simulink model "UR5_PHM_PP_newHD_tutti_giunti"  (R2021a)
settings: Solver=ode14x  StartTime=0.0  StopTime=Sim.time  FixedStep=Sim.dt  MaxStep=Sim.dt  RelTol=1e-3  EnableMultiTasking=on
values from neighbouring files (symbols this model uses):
  alpha_n = 0.98*pi/180    (= 0.0171042266695)    [parameters.m]
  alpha_t = 30*pi/180    (= 0.523598775598)    [parameters.m]
  alpha_TTS = 0    [parameters.m]
  alpha_Tw_L = -6.9e-4    (= -0.00069)    [parameters.m]
  alpha_Tw_R = 3.9e-3    (= 0.0039)    [parameters.m]
  Beta_TTS = 0    [parameters.m]
  c1 = 1e-2    (= 0.01)    [parameters.m]
  c2 = 1e-2    (= 0.01)    [parameters.m]
  c3 = 1e-2    (= 0.01)    [parameters.m]
  c4 = 1e-2    (= 0.01)    [parameters.m]
  c5 = 1e-2    (= 0.01)    [parameters.m]
  c6 = 1e-2    (= 0.01)    [parameters.m]
  Cb1 = 1.8e3    (= 1800)    [parameters.m]
  Cb2 = 1.8e3    (= 1800)    [parameters.m]
  Cb3 = 1.8e3    (= 1800)    [parameters.m]
  Cb4 = 1.8e3    (= 1800)    [parameters.m]
  Cb5 = 1.8e3    (= 1800)    [parameters.m]
  Cb6 = 1.8e3    (= 1800)    [parameters.m]
  Cth_housing = 153.90    (= 153.9)    [parameters.m]
  Cth_w = 74.20    (= 74.2)    [parameters.m]
  dt_PP = 0.05    [parameters.m]
  Fric1 = [fc_1/2 1e1 fc_1 fv_1]    [parameters.m]
  Fric2 = [fc_2/2 1e1 fc_2 fv_2]    [parameters.m]
  Fric3 = [fc_3/2 1e1 fc_3 fv_3]    [parameters.m]
  Fric4 = [fc_4/2 1e1 fc_4 fv_4]    [parameters.m]
  Fric5 = [fc_5/2 1e1 fc_5 fv_5]    [parameters.m]
  Fric6 = [fc_6/2 1e1 fc_6 fv_6]    [parameters.m]
  Hth_housing = 0.30    (= 0.3)    [parameters.m]
  Hth_w = 1.14    [parameters.m]
  I_actual = I_actual(1:10,:)    [trajcutting.m]
  J_CS1 = 7.12e-5    (= 7.12e-05)    [parameters.m]
  J_CS2 = 7.12e-5    (= 7.12e-05)    [parameters.m]
  J_CS3 = 7.12e-5    (= 7.12e-05)    [parameters.m]
  J_CS4 = 6e-6    (= 6e-06)    [parameters.m]
  J_CS5 = 6e-6    (= 6e-06)    [parameters.m]
  J_CS6 = 6e-6    (= 6e-06)    [parameters.m]
  J_FS1 = 1.62e-7    (= 1.62e-07)    [parameters.m]
  J_FS2 = 1.62e-7    (= 1.62e-07)    [parameters.m]
  J_FS3 = 1.62e-7    (= 1.62e-07)    [parameters.m]
  J_FS4 = 4.97e-8    (= 4.97e-08)    [parameters.m]
  J_FS5 = 4.97e-8    (= 4.97e-08)    [parameters.m]
  J_FS6 = 4.97e-8    (= 4.97e-08)    [parameters.m]
  J_WG1 = 3.56e-5    (= 3.56e-05)    [parameters.m]
  J_WG2 = 3.56e-5    (= 3.56e-05)    [parameters.m]
  J_WG3 = 3.56e-5    (= 3.56e-05)    [parameters.m]
  J_WG4 = 3e-6    (= 3e-06)    [parameters.m]
  J_WG5 = 3e-6    (= 3e-06)    [parameters.m]
  J_WG6 = 3e-6    (= 3e-06)    [parameters.m]
  K_i = 1    [parameters.m]
  K_p = 1    [parameters.m]
  K_torsCS1 = 4.78e6    (= 4780000)    [parameters.m]
  K_torsCS2 = 4.78e6    (= 4780000)    [parameters.m]
  K_torsCS3 = 4.78e6    (= 4780000)    [parameters.m]
  K_torsCS4 = 1.06e6    (= 1060000)    [parameters.m]
  K_torsCS5 = 1.06e6    (= 1060000)    [parameters.m]
  K_torsCS6 = 1.06e6    (= 1060000)    [parameters.m]
  K_torsWG1 = 9.56e5    (= 956000)    [parameters.m]
  K_torsWG2 = 9.56e5    (= 956000)    [parameters.m]
  K_torsWG3 = 9.56e5    (= 956000)    [parameters.m]
  K_torsWG4 = 1.84e5    (= 184000)    [parameters.m]
  K_torsWG5 = 1.84e5    (= 184000)    [parameters.m]
  K_torsWG6 = 1.84e5    (= 184000)    [parameters.m]
  K_v = 1    [parameters.m]
  Kb1 = 0.51e8    (= 51000000)    [parameters.m]
  Kb2 = 0.51e8    (= 51000000)    [parameters.m]
  Kb3 = 0.51e8    (= 51000000)    [parameters.m]
  Kb4 = 1.98e7    (= 19800000)    [parameters.m]
  Kb5 = 1.98e7    (= 19800000)    [parameters.m]
  Kb6 = 1.98e7    (= 19800000)    [parameters.m]
  Km1 = 1.2e9    (= 1200000000)    [parameters.m]
  Km2 = 1.2e9    (= 1200000000)    [parameters.m]
  Km3 = 1.2e9    (= 1200000000)    [parameters.m]
  Km4 = 5.55e8    (= 555000000)    [parameters.m]
  Km5 = 5.55e8    (= 555000000)    [parameters.m]
  Km6 = 5.55e8    (= 555000000)    [parameters.m]
  Kt1 = 0.96e5    (= 96000)    [parameters.m]
  Kt2 = 0.96e5    (= 96000)    [parameters.m]
  Kt3 = 0.96e5    (= 96000)    [parameters.m]
  Kt4 = 1.15e4    (= 11500)    [parameters.m]
  Kt5 = 1.15e4    (= 11500)    [parameters.m]
  Kt6 = 1.15e4    (= 11500)    [parameters.m]
  L = Motor.L_2/2    [parameters.m]
  m2 = polyfit(Temp(:,2),pBn_UR5_f_Temp(:,2),1)    [parameters.m]
  mb2 = polyfit(Temp(:,8),pBn_UR5_f_Temp(:,8),1)    [parameters.m]
  pickTime = t_pick(traj)    [parameters.m]
  placeTime = t_place(traj)    [parameters.m]
  q0 = q_target(1,:)    [testlaw_PP.m]
  q_CS01 = x(6)    [parameters.m]
  q_CS02 = x(6)    [parameters.m]
  q_CS03 = x(6)    [parameters.m]
  q_CS04 = x(6)    [parameters.m]
  q_CS05 = x(6)    [parameters.m]
  q_CS06 = x(6)    [parameters.m]
  q_WG01 = x(1)    [parameters.m]
  q_WG02 = x(1)    [parameters.m]
  q_WG03 = x(1)    [parameters.m]
  q_WG04 = x(1)    [parameters.m]
  q_WG05 = x(1)    [parameters.m]
  q_WG06 = x(1)    [parameters.m]
  quant_i = [Motor.imax1 Motor.imax2      Motor.imax3 Motor.imax4 Motor.imax5 Motor.imax6]/2^16    [parameters.m]
  R = Motor.R_2/2    [parameters.m]
  rg1 = 0.028    [parameters.m]
  rg2 = 0.028    [parameters.m]
  rg3 = 0.028    [parameters.m]
  rg4 = 0.0155    [parameters.m]
  rg5 = 0.0155    [parameters.m]
  rg6 = 0.0155    [parameters.m]
  sigma_p = 444.29    [parameters.m]
  sigma_v = 2*pi*1000    (= 6283.18530718)    [parameters.m]
  stiff_red = 1    [parameters.m]
  T_0 = Sim.temp    [parameters.m]
  T_switch = 1e-4    (= 0.0001)    [parameters.m]
  tau_i = 1/(fc_i*2*pi)    (= 7.95774715459e-05)    [parameters.m]
  U_s = 48    [parameters.m]
  var_i = 1e-1*[.0167 .0184 .0144 .0016      .0011 .0007]    [parameters.m]
  var_p = 1e-6*[.0943 .3877      .3478 .5436 .3400 .2081]    [parameters.m]
  var_v = 1e-4*[.0738 .1452      .1564 .4623 .1824 .0917]    [parameters.m]
  Wf_TTS_0 = 0    [parameters.m]
  Wf_TTS_ONOFF = 0    [parameters.m]
  x2_01 = x(3)    [parameters.m]
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undefined symbols (not defined in the file or in its folder): deg, Driver1, Driver2, Driver3, Driver4, Driver5, Driver6, elseif, geom, Ground, J1, J2, J3, J4, J5, J6, kg, L1, L2, L3, L4, L5, L6, LINK0, LINK1, LINK2, LINK3, LINK4, LINK5, LINK6, m, Motor, N, payload, ROBOTIQ_FT, s, Sim, Tool, X, Y, Z
libraries: sm_lib x35, nesl_utility x30, simulink x23, simulink_extras x11, spsTriangleGeneratorLib x6
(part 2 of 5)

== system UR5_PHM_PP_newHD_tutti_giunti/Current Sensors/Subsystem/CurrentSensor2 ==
  qm2 : Inport
  i2 [a,b,c] : Inport  Port=2
  Demux1 : Demux  Outputs=3
  Mux1 : Mux  Inputs=3
  Noise : UniformRandomNumber  Minimum=-var_i(2)  Maximum=var_i(2)  SampleTime=1/50
  Park Trnasform : Subsystem
  "Quantizer " : Quantizer  QuantizationInterval=quant_i(2)
  Sum : Sum  Inputs=|++
  Transfer Fcn : TransferFcn  Numerator=[K_i]  Denominator=[tau_i 1]
  Transfer Fcn1 : TransferFcn  Numerator=[K_i]  Denominator=[tau_i 1]
  Transfer Fcn2 : TransferFcn  Numerator=[K_i]  Denominator=[tau_i 1]
  "Zero-Order Hold " : ZeroOrderHold  SampleTime=1e-6
  i2 [dq0] : Outport
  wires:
  i2 [a,b,c]/1 -> Demux1/1
  Park Trnasform/1(i[d,q,0]) -> i2 [dq0]/1
  qm2/1 -> Park Trnasform/2(qm2)
  Noise/1 -> Sum/2
  "Quantizer "/1 -> Park Trnasform/1(i[a,b,c])
  "Zero-Order Hold "/1 -> "Quantizer "/1
  Sum/1 -> "Zero-Order Hold "/1
  Mux1/1 -> Sum/1
  Demux1/1 -> Transfer Fcn/1
  Demux1/2 -> Transfer Fcn1/1
  Demux1/3 -> Transfer Fcn2/1
  Transfer Fcn/1 -> Mux1/1
  Transfer Fcn1/1 -> Mux1/2
  Transfer Fcn2/1 -> Mux1/3

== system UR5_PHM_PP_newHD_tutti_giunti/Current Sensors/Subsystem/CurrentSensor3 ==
  i3 : Inport
  Noise : UniformRandomNumber  Minimum=-var_i(3)  Maximum=var_i(3)  SampleTime=1/50
  "Quantizer " : Quantizer  QuantizationInterval=quant_i(3)
  Sum : Sum  Inputs=|++
  Transfer Fcn (with initial outputs) : simulink_extras/Additional Linear/Transfer Fcn (with initial outputs)  N=[K_i]  D=[tau_i 1]  Y0=I_actual(1,3)  U0=I_actual(1,3)
  "Zero-Order Hold " : ZeroOrderHold  SampleTime=1e-6
  i3FB : Outport
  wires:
  Noise/1 -> Sum/2
  "Quantizer "/1 -> i3FB/1
  "Zero-Order Hold "/1 -> "Quantizer "/1
  Sum/1 -> "Zero-Order Hold "/1
  Transfer Fcn (with initial outputs)/1 -> Sum/1
  i3/1 -> Transfer Fcn (with initial outputs)/1

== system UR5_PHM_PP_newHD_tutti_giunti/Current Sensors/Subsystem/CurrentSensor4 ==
  i4 : Inport
  Noise : UniformRandomNumber  Minimum=-var_i(4)  Maximum=var_i(4)  SampleTime=1/50
  "Quantizer " : Quantizer  QuantizationInterval=quant_i(4)
  Sum : Sum  Inputs=|++
  Transfer Fcn (with initial outputs) : simulink_extras/Additional Linear/Transfer Fcn (with initial outputs)  N=[K_i]  D=[tau_i 1]  Y0=I_actual(1,4)  U0=I_actual(1,4)
  "Zero-Order Hold " : ZeroOrderHold  SampleTime=1e-6
  i4FB : Outport
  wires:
  Noise/1 -> Sum/2
  "Quantizer "/1 -> i4FB/1
  "Zero-Order Hold "/1 -> "Quantizer "/1
  Sum/1 -> "Zero-Order Hold "/1
  Transfer Fcn (with initial outputs)/1 -> Sum/1
  i4/1 -> Transfer Fcn (with initial outputs)/1

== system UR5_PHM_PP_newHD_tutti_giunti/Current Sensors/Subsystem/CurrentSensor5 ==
  i5 : Inport
  Noise : UniformRandomNumber  Minimum=-var_i(5)  Maximum=var_i(5)  SampleTime=1/50
  "Quantizer " : Quantizer  QuantizationInterval=quant_i(5)
  Sum : Sum  Inputs=|++
  Transfer Fcn (with initial outputs) : simulink_extras/Additional Linear/Transfer Fcn (with initial outputs)  N=[K_i]  D=[tau_i 1]  Y0=I_actual(1,5)  U0=I_actual(1,5)
  "Zero-Order Hold " : ZeroOrderHold  SampleTime=1e-6
  i5FB : Outport
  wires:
  Noise/1 -> Sum/2
  "Quantizer "/1 -> i5FB/1
  "Zero-Order Hold "/1 -> "Quantizer "/1
  Sum/1 -> "Zero-Order Hold "/1
  Transfer Fcn (with initial outputs)/1 -> Sum/1
  i5/1 -> Transfer Fcn (with initial outputs)/1

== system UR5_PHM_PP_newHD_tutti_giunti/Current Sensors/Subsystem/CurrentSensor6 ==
  i6 : Inport
  Noise : UniformRandomNumber  Minimum=-var_i(6)  Maximum=var_i(6)  SampleTime=1/50
  "Quantizer " : Quantizer  QuantizationInterval=quant_i(6)
  Sum : Sum  Inputs=|++
  Transfer Fcn (with initial outputs) : simulink_extras/Additional Linear/Transfer Fcn (with initial outputs)  N=[K_i]  D=[tau_i 1]  Y0=I_actual(1,6)  U0=I_actual(1,6)
  "Zero-Order Hold " : ZeroOrderHold  SampleTime=1e-6
  i6FB : Outport
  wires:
  "Quantizer "/1 -> i6FB/1
  Noise/1 -> Sum/2
  "Zero-Order Hold "/1 -> "Quantizer "/1
  Sum/1 -> "Zero-Order Hold "/1
  Transfer Fcn (with initial outputs)/1 -> Sum/1
  i6/1 -> Transfer Fcn (with initial outputs)/1

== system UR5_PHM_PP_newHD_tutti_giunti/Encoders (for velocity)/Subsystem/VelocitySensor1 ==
  qdm1 : Inport
  Noise : UniformRandomNumber  Minimum=-var_v(1)  Maximum=var_v(1)  SampleTime=1/5
  "Quantizer " : Quantizer  QuantizationInterval=quant_v
  Sum : Sum  Inputs=|++
  Transfer Fcn2 : TransferFcn  Numerator=[K_v]  Denominator=[1/sigma_v^2 2*zeta_v/sigma_v 1]
  "Zero-Order Hold " : ZeroOrderHold  SampleTime=1e-6
  qdmFB : Outport
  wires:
  qdm1/1 -> Transfer Fcn2/1
  Noise/1 -> Sum/2
  "Quantizer "/1 -> qdmFB/1
  "Zero-Order Hold "/1 -> "Quantizer "/1
  Sum/1 -> "Zero-Order Hold "/1
  Transfer Fcn2/1 -> Sum/1

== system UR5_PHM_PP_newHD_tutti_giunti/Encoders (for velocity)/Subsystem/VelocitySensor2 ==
  qdm2 : Inport
  Noise : UniformRandomNumber  Minimum=-var_v(2)  Maximum=var_v(2)  SampleTime=1/5
  "Quantizer " : Quantizer  QuantizationInterval=quant_v
  Sum : Sum  Inputs=|++
  Transfer Fcn2 : TransferFcn  Numerator=[K_v]  Denominator=[1/sigma_v^2 2*zeta_v/sigma_v 1]
  "Zero-Order Hold " : ZeroOrderHold  SampleTime=1e-6
  qdmFB2 : Outport
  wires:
  Noise/1 -> Sum/2
  "Quantizer "/1 -> qdmFB2/1
  "Zero-Order Hold "/1 -> "Quantizer "/1
  Sum/1 -> "Zero-Order Hold "/1
  qdm2/1 -> Transfer Fcn2/1
  Transfer Fcn2/1 -> Sum/1

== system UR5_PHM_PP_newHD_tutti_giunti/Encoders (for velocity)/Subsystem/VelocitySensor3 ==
  qdm3 : Inport
  Noise : UniformRandomNumber  Minimum=-var_v(3)  Maximum=var_v(3)  SampleTime=1/5
  "Quantizer " : Quantizer  QuantizationInterval=quant_v
  Sum : Sum  Inputs=|++
  Transfer Fcn2 : TransferFcn  Numerator=[K_v]  Denominator=[1/sigma_v^2 2*zeta_v/sigma_v 1]
  "Zero-Order Hold " : ZeroOrderHold  SampleTime=1e-6
  qdm3FB : Outport
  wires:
  Noise/1 -> Sum/2
  "Quantizer "/1 -> qdm3FB/1
  "Zero-Order Hold "/1 -> "Quantizer "/1
  Sum/1 -> "Zero-Order Hold "/1
  Transfer Fcn2/1 -> Sum/1
  qdm3/1 -> Transfer Fcn2/1

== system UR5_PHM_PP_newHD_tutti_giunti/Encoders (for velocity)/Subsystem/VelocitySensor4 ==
  qdm4 : Inport
  Noise : UniformRandomNumber  Minimum=-var_v(4)  Maximum=var_v(4)  SampleTime=1/5
  "Quantizer " : Quantizer  QuantizationInterval=quant_v
  Sum : Sum  Inputs=|++
  Transfer Fcn2 : TransferFcn  Numerator=[K_v]  Denominator=[1/sigma_v^2 2*zeta_v/sigma_v 1]
  "Zero-Order Hold " : ZeroOrderHold  SampleTime=1e-6
  qdm4FB : Outport
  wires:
  Noise/1 -> Sum/2
  "Quantizer "/1 -> qdm4FB/1
  "Zero-Order Hold "/1 -> "Quantizer "/1
  Sum/1 -> "Zero-Order Hold "/1
  Transfer Fcn2/1 -> Sum/1
  qdm4/1 -> Transfer Fcn2/1

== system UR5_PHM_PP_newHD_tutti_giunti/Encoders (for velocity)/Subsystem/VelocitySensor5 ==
  qdm5 : Inport
  Noise : UniformRandomNumber  Minimum=-var_v(5)  Maximum=var_v(5)  SampleTime=1/5
  "Quantizer " : Quantizer  QuantizationInterval=quant_v
  Sum : Sum  Inputs=|++
  Transfer Fcn2 : TransferFcn  Numerator=[K_v]  Denominator=[1/sigma_v^2 2*zeta_v/sigma_v 1]
  "Zero-Order Hold " : ZeroOrderHold  SampleTime=1e-6
  qdm5FB : Outport
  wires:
  Noise/1 -> Sum/2
  "Quantizer "/1 -> qdm5FB/1
  "Zero-Order Hold "/1 -> "Quantizer "/1
  Sum/1 -> "Zero-Order Hold "/1
  Transfer Fcn2/1 -> Sum/1
  qdm5/1 -> Transfer Fcn2/1

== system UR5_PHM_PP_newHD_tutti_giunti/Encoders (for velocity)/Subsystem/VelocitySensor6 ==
  qdm6 : Inport
  Noise : UniformRandomNumber  Minimum=-var_v(6)  Maximum=var_v(6)  SampleTime=1/5
  "Quantizer " : Quantizer  QuantizationInterval=quant_v
  Sum : Sum  Inputs=|++
  Transfer Fcn2 : TransferFcn  Numerator=[K_v]  Denominator=[1/sigma_v^2 2*zeta_v/sigma_v 1]
  "Zero-Order Hold " : ZeroOrderHold  SampleTime=1e-6
  qdm6FB : Outport
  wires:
  Noise/1 -> Sum/2
  "Quantizer "/1 -> qdm6FB/1
  "Zero-Order Hold "/1 -> "Quantizer "/1
  Sum/1 -> "Zero-Order Hold "/1
  Transfer Fcn2/1 -> Sum/1
  qdm6/1 -> Transfer Fcn2/1

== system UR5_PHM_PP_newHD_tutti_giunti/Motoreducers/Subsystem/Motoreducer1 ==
  q,qd,qdd : Inport
  Vset : Inport  Port=2
  DC Monophase Motor : Subsystem
  Demux : Demux  Outputs=3
  Demux1 : Demux  Outputs=3
  Gain : Gain  Gain=Motor.tau
  Gain1 : Gain  Gain=Motor.tau
  Gearbox : Subsystem
  New Gearbox's model : Subsystem
  Sum : Sum  Inputs=-+|
  Sum1 : Sum  Inputs=-+|
  Terminator : Terminator
  Terminator1 : Terminator
  Tu : Outport
  i : Outport  Port=2
  qm,qdm,qddm : Outport  Port=3
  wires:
  New Gearbox's model/2(C2) -> Gearbox/1(C)
  Sum1/1 -> New Gearbox's model/3(Delta_qd)
  Gain1/1 -> Sum1/1
  DC Monophase Motor/2(qm,qdm,qddm) -> qm,qdm,qddm/1, Demux/1
  Sum/1 -> New Gearbox's model/1(Delta_q)
  Demux/2 -> New Gearbox's model/4(qdm), Sum1/2
  Demux/3 -> Terminator1/1
  Demux1/1 -> [q], Gain/1
  Demux1/3 -> Terminator/1
  DC Monophase Motor/1(i) -> i/1
  Demux/1 -> Sum/2, New Gearbox's model/2(qm)
  Demux1/2 -> [qd], Gain1/1
  Vset/1 -> DC Monophase Motor/1(Vset)
  Gearbox/1(Tu) -> Tu/1  "Tu_j1"
  Gain/1 -> Sum/1
  q,qd,qdd/1 -> Demux1/1
  [qd] -> Gearbox/2(qd)
  [q] -> New Gearbox's model/5(q)
  [qd] -> New Gearbox's model/6(qd)
  New Gearbox's model/1(C1) -> DC Monophase Motor/2(C)

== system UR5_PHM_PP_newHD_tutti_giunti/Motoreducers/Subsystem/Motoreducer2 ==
  q,qd,qdd : Inport
  Vset : Inport  Port=2
  BLAC : Subsystem
  Constant : Constant  Value=Sim.temp
  Demux : Demux  Outputs=3
  Demux1 : Demux  Outputs=3
  Gain : Gain  Gain=Motor.tau
  Gain1 : Gain  Gain=Motor.tau
  Gearbox : Subsystem
  New Gearbox's Model : Subsystem
  Scope : Scope
  Scope1 : Scope
  Sum : Sum  Inputs=-+|
  Sum1 : Sum  Inputs=-+|
  Terminator : Terminator
  Terminator1 : Terminator
  Windings temperature : Subsystem
  Tu : Outport
  i[a.b.c] : Outport  Port=2
  qm,qdm,qddm : Outport  Port=3
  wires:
  Windings temperature/1(Tw [°C]) -> BLAC/2(T_w [°C])
  BLAC/3(W_joule[W]) -> Windings temperature/1(W_joule [W])
  Vset/1 -> BLAC/1(V[ao,bo,co])
  Constant/1 -> Windings temperature/2(T_ext [°C])
  BLAC/1(i[a,b,c]) -> i[a.b.c]/1
  q,qd,qdd/1 -> Demux1/1
  Demux1/2 -> [qd], Gain1/1
  Demux1/3 -> Terminator/1
  Gain1/1 -> Sum1/1
  BLAC/2(qm,qdm,qddm) -> Demux/1, qm,qdm,qddm/1
  Demux/1 -> New Gearbox's Model/2(qm), Sum/2
  Gain/1 -> Sum/1
  Sum/1 -> Scope/1, New Gearbox's Model/1(Delta_q)  "Delta_q_j2"
  Sum1/1 -> New Gearbox's Model/3(Delta_qd)
  Demux/3 -> Terminator1/1
  Demux/2 -> New Gearbox's Model/4(qdm), Sum1/2
  Demux1/1 -> [q], Gain/1
  [qd] -> Gearbox/2(qd)
  Gearbox/1(Tu) -> Tu/1  "Tu_j2"
  Windings temperature/2(Th [°C]) -> Gearbox/3(Th [°C])
  New Gearbox's Model/2(C2) -> Scope1/1, Gearbox/1(C)
  [q] -> New Gearbox's Model/5(q)
  New Gearbox's Model/1(C1) -> BLAC/3(C)
  [qd] -> New Gearbox's Model/6(qd)

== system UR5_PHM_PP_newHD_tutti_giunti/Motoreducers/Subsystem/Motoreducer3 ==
  q,qd,qdd : Inport
  Vset : Inport  Port=2
  DC Monophase Motor3 : Subsystem
  Demux4 : Demux  Outputs=3
  Demux5 : Demux  Outputs=3
  Gain4 : Gain  Gain=Motor.tau
  Gain5 : Gain  Gain=Motor.tau
  Gearbox3 : Subsystem
  New Gearbox's Model : Subsystem
  Sum4 : Sum  Inputs=-+|
  Sum5 : Sum  Inputs=-+|
  Terminator4 : Terminator
  Terminator5 : Terminator
  Tu : Outport
  i : Outport  Port=2
  qm,qdm,qddm : Outport  Port=3
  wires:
  Gain4/1 -> Sum4/1
  Sum5/1 -> New Gearbox's Model/4(Delta_qd)
  New Gearbox's Model/2(Tu) -> Gearbox3/1(C)
  DC Monophase Motor3/2(qm,qdm,qddm) -> qm,qdm,qddm/1, Demux4/1
  Demux5/3 -> Terminator4/1
  Demux5/2 -> [qd], Gain5/1
  Demux4/2 -> New Gearbox's Model/3(qdm), Sum5/2
  Demux4/3 -> Terminator5/1
  Sum4/1 -> New Gearbox's Model/1(Delta_q)
  [qd] -> Gearbox3/2(qd)
  DC Monophase Motor3/1(i) -> i/1
  Demux5/1 -> [q], Gain4/1
  Vset/1 -> DC Monophase Motor3/1(Vset)
  q,qd,qdd/1 -> Demux5/1
  Gain5/1 -> Sum5/1
  Gearbox3/1(Tu) -> Tu/1  "Tu_j3"
  Demux4/1 -> New Gearbox's Model/2(qm), Sum4/2
  [q] -> New Gearbox's Model/5(q)
  [qd] -> New Gearbox's Model/6(qd)
  New Gearbox's Model/1(C1) -> DC Monophase Motor3/2(C)

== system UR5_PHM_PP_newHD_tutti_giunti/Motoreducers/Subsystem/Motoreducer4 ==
  q,qd,qdd : Inport
  Vset : Inport  Port=2
  DC Monophase Motor4 : Subsystem
  Demux6 : Demux  Outputs=3
  Demux7 : Demux  Outputs=3
  Gain6 : Gain  Gain=Motor.tau
  Gain7 : Gain  Gain=Motor.tau
  Gearbox4 : Subsystem
  New Gearbox's Model : Subsystem
  Sum6 : Sum  Inputs=-+|
  Sum7 : Sum  Inputs=-+|
  Terminator6 : Terminator
  Terminator7 : Terminator
  Tu : Outport
  i : Outport  Port=2
  qm,qdm,qddm : Outport  Port=3
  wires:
  Demux7/2 -> [qd], Gain7/1
  DC Monophase Motor4/2(qm,qdm,qddm) -> qm,qdm,qddm/1, Demux6/1
  Gain7/1 -> Sum7/1
  Sum6/1 -> New Gearbox's Model/1(Delta_q)
  [qd] -> Gearbox4/2(qd)
  Demux6/2 -> New Gearbox's Model/3(qdm), Sum7/2
  New Gearbox's Model/2(C2) -> Gearbox4/1(C)
  Gain6/1 -> Sum6/1
  Demux7/3 -> Terminator6/1
  Demux6/1 -> New Gearbox's Model/2(qm), Sum6/2
  Demux7/1 -> Gain6/1, [q]
  DC Monophase Motor4/1(i) -> i/1
  Sum7/1 -> New Gearbox's Model/4(Delta_qd)
  q,qd,qdd/1 -> Demux7/1
  Vset/1 -> DC Monophase Motor4/1(Vset)
  Demux6/3 -> Terminator7/1
  Gearbox4/1(Tu) -> Tu/1  "Tu_j4"
  [q] -> New Gearbox's Model/5(q)
  [qd] -> New Gearbox's Model/6(qd)
  New Gearbox's Model/1(C1) -> DC Monophase Motor4/2(C)

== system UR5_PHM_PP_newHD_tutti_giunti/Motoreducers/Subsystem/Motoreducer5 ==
  q,qd,qdd : Inport
  Vset : Inport  Port=2
  DC Monophase Motor5 : Subsystem
  Demux8 : Demux  Outputs=3
  Demux9 : Demux  Outputs=3
  Gain8 : Gain  Gain=Motor.tau
  Gain9 : Gain  Gain=Motor.tau
  Gearbox5 : Subsystem
  New Gearbox's Model : Subsystem
  Sum8 : Sum  Inputs=-+|
  Sum9 : Sum  Inputs=-+|
  Terminator8 : Terminator
  Terminator9 : Terminator
  Tu : Outport
  i : Outport  Port=2
  qm,qdm,qddm : Outport  Port=3
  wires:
  Demux9/3 -> Terminator8/1
  Demux8/1 -> New Gearbox's Model/2(qm), Sum8/2
  Gain8/1 -> Sum8/1
  New Gearbox's Model/2(C2) -> Gearbox5/1(C)
  Demux8/3 -> Terminator9/1
  Demux8/2 -> New Gearbox's Model/3(qdm), Sum9/2
  Gain9/1 -> Sum9/1
  Sum9/1 -> New Gearbox's Model/4(Delta_qd)
  Sum8/1 -> New Gearbox's Model/1(Delta_q)
  Demux9/1 -> [q], Gain8/1
  Vset/1 -> DC Monophase Motor5/1(Vset)
  Demux9/2 -> [qd], Gain9/1
  DC Monophase Motor5/2(qm,qdm,qddm) -> qm,qdm,qddm/1, Demux8/1
  q,qd,qdd/1 -> Demux9/1
  [qd] -> Gearbox5/2(qd)
  DC Monophase Motor5/1(i) -> i/1
  Gearbox5/1(Tu) -> Tu/1  "Tu_j5"
  [q] -> New Gearbox's Model/5(q)
  [qd] -> New Gearbox's Model/6(qd)
  New Gearbox's Model/1(C1) -> DC Monophase Motor5/2(C)

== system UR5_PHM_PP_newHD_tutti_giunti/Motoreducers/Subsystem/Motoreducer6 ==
  q,qd,qdd : Inport
  Vset : Inport  Port=2
  DC Monophase Motor6 : Subsystem
  Demux10 : Demux  Outputs=3
  Demux11 : Demux  Outputs=3
  Gain10 : Gain  Gain=Motor.tau
  Gain11 : Gain  Gain=Motor.tau
  Gearbox6 : Subsystem
  New  Gearbox's Model : Subsystem
  Sum10 : Sum  Inputs=-+|
  Sum11 : Sum  Inputs=-+|
  Terminator10 : Terminator
  Terminator11 : Terminator
  Tu : Outport
  i : Outport  Port=2
  qm,qdm,qddm : Outport  Port=3
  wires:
  Vset/1 -> DC Monophase Motor6/1(Vset)
  q,qd,qdd/1 -> Demux11/1
  DC Monophase Motor6/1(i) -> i/1
  Demux11/1 -> Gain10/1, [q]
  Gain10/1 -> Sum10/1
  Demux10/1 -> New  Gearbox's Model/2(qm), Sum10/2
  Demux11/2 -> [qd], Gain11/1
  Sum11/1 -> New  Gearbox's Model/4(Delta_qd)
  [qd] -> Gearbox6/2(qd)
  Sum10/1 -> New  Gearbox's Model/1(Delta_q)
  Demux10/2 -> New  Gearbox's Model/3(qdm), Sum11/2
  Demux10/3 -> Terminator11/1
  New  Gearbox's Model/2(C2) -> Gearbox6/1(C)
  DC Monophase Motor6/2(qm,qdm,qddm) -> qm,qdm,qddm/1, Demux10/1
  Demux11/3 -> Terminator10/1
  Gain11/1 -> Sum11/1
  Gearbox6/1(Tu) -> Tu/1  "Tu_j6"
  [q] -> New  Gearbox's Model/5(q)
  [qd] -> New  Gearbox's Model/6(qd)
  New  Gearbox's Model/1(C1) -> DC Monophase Motor6/2(C)

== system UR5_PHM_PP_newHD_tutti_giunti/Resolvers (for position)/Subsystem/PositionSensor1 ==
  q1 : Inport
  Noise : UniformRandomNumber  Minimum=-var_p(1)  Maximum=var_p(1)  SampleTime=1/4
  "Quantizer " : Quantizer  QuantizationInterval=quant_p
  Sum : Sum  Inputs=|++
  Transfer Fcn (with initial outputs)2 : simulink_extras/Additional Linear/Transfer Fcn (with initial outputs)  N=[K_p]  D=[1/sigma_p^2 2*zeta_p/sigma_p 1]  Y0=q0(1)  U0=q0(1)
  "Zero-Order Hold " : ZeroOrderHold  SampleTime=1e-6
  q1FB : Outport
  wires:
  Noise/1 -> Sum/2
  "Quantizer "/1 -> q1FB/1
  "Zero-Order Hold "/1 -> "Quantizer "/1
  Sum/1 -> "Zero-Order Hold "/1
  Transfer Fcn (with initial outputs)2/1 -> Sum/1
  q1/1 -> Transfer Fcn (with initial outputs)2/1

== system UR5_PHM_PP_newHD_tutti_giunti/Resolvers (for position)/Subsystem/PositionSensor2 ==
  q2 : Inport
  Noise : UniformRandomNumber  Minimum=-var_p(2)  Maximum=var_p(2)  SampleTime=1/4
  "Quantizer " : Quantizer  QuantizationInterval=quant_p
  Sum : Sum  Inputs=|++
  Transfer Fcn (with initial outputs)2 : simulink_extras/Additional Linear/Transfer Fcn (with initial outputs)  N=[K_p]  D=[1/sigma_p^2 2*zeta_p/sigma_p 1]  Y0=q0(2)  U0=q0(2)
  "Zero-Order Hold " : ZeroOrderHold  SampleTime=1e-6
  q2FB : Outport
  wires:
  "Quantizer "/1 -> q2FB/1
  "Zero-Order Hold "/1 -> "Quantizer "/1
  Sum/1 -> "Zero-Order Hold "/1
  Transfer Fcn (with initial outputs)2/1 -> Sum/1
  q2/1 -> Transfer Fcn (with initial outputs)2/1
  Noise/1 -> Sum/2

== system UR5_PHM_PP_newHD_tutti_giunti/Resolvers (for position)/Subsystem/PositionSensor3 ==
  q3 : Inport
  Noise : UniformRandomNumber  Minimum=-var_p(3)  Maximum=var_p(3)  SampleTime=1/4
  "Quantizer " : Quantizer  QuantizationInterval=quant_p
  Sum : Sum  Inputs=|++
  Transfer Fcn (with initial outputs)2 : simulink_extras/Additional Linear/Transfer Fcn (with initial outputs)  N=[K_p]  D=[1/sigma_p^2 2*zeta_p/sigma_p 1]  Y0=q0(3)  U0=q0(3)
  "Zero-Order Hold " : ZeroOrderHold  SampleTime=1e-6
  q3FB : Outport
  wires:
  Sum/1 -> "Zero-Order Hold "/1
  "Zero-Order Hold "/1 -> "Quantizer "/1
  "Quantizer "/1 -> q3FB/1
  Noise/1 -> Sum/2
  q3/1 -> Transfer Fcn (with initial outputs)2/1
  Transfer Fcn (with initial outputs)2/1 -> Sum/1

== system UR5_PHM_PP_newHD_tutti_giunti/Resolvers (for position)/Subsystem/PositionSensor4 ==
  q4 : Inport
  Noise : UniformRandomNumber  Minimum=-var_p(4)  Maximum=var_p(4)  SampleTime=1/4
  "Quantizer " : Quantizer  QuantizationInterval=quant_p
  Sum : Sum  Inputs=|++
  Transfer Fcn (with initial outputs)2 : simulink_extras/Additional Linear/Transfer Fcn (with initial outputs)  N=[K_p]  D=[1/sigma_p^2 2*zeta_p/sigma_p 1]  Y0=q0(4)  U0=q0(4)
  "Zero-Order Hold " : ZeroOrderHold  SampleTime=1e-6
  q4FB : Outport
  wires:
  Noise/1 -> Sum/2
  "Quantizer "/1 -> q4FB/1
  "Zero-Order Hold "/1 -> "Quantizer "/1
  Sum/1 -> "Zero-Order Hold "/1
  q4/1 -> Transfer Fcn (with initial outputs)2/1
  Transfer Fcn (with initial outputs)2/1 -> Sum/1

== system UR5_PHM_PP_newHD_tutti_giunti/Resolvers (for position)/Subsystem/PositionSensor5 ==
  q5 : Inport
  Noise : UniformRandomNumber  Minimum=-var_p(5)  Maximum=var_p(5)  SampleTime=1/4
  "Quantizer " : Quantizer  QuantizationInterval=quant_p
  Sum : Sum  Inputs=|++
  Transfer Fcn (with initial outputs)2 : simulink_extras/Additional Linear/Transfer Fcn (with initial outputs)  N=[K_p]  D=[1/sigma_p^2 2*zeta_p/sigma_p 1]  Y0=q0(5)  U0=q0(5)
  "Zero-Order Hold " : ZeroOrderHold  SampleTime=1e-6
  q5FB : Outport
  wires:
  Sum/1 -> "Zero-Order Hold "/1
  "Zero-Order Hold "/1 -> "Quantizer "/1
  "Quantizer "/1 -> q5FB/1
  Noise/1 -> Sum/2
  q5/1 -> Transfer Fcn (with initial outputs)2/1
  Transfer Fcn (with initial outputs)2/1 -> Sum/1

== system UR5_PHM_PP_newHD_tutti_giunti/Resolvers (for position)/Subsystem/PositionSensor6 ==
  q6 : Inport
  Noise : UniformRandomNumber  Minimum=-var_p(6)  Maximum=var_p(6)  SampleTime=1/4
  "Quantizer " : Quantizer  QuantizationInterval=quant_p
  Sum : Sum  Inputs=|++
  Transfer Fcn (with initial outputs)2 : simulink_extras/Additional Linear/Transfer Fcn (with initial outputs)  N=[K_p]  D=[1/sigma_p^2 2*zeta_p/sigma_p 1]  Y0=q0(6)  U0=q0(6)
  "Zero-Order Hold " : ZeroOrderHold  SampleTime=1e-6
  q6FB : Outport
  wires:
  Noise/1 -> Sum/2
  "Quantizer "/1 -> q6FB/1
  "Zero-Order Hold "/1 -> "Quantizer "/1
  Sum/1 -> "Zero-Order Hold "/1
  Transfer Fcn (with initial outputs)2/1 -> Sum/1
  q6/1 -> Transfer Fcn (with initial outputs)2/1

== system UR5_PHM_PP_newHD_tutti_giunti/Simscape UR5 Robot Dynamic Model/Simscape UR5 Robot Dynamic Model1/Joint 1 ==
  T1 : Inport
  A_01*E_01 : sm_lib/Frames and Transforms/Rigid Transform  TranslationMethod=None  TranslationStandardOffset=0  TranslationLengthUnit=mm  TranslationStandardAxis=+Z  TranslationCartesianOffset=A01t  TranslationROffset=0  TranslationROffsetUnits=m  TranslationZOffset=0  TranslationZOffsetUnits=m  TranslationThetaOffset=0  TranslationThetaOffsetUnits=deg  RotationMethod=RotationMatrix  RotationAngleUnits=deg  RotationStandardAxis=+Z  RotationAngle=0.0  RotationArbitraryAxis=[0 0 1]  FollAlignAxisA=+X  BaseAlignAxisA=+Y  FollAlignAxisB=+Y  BaseAlignAxisB=+Z  RotationSequenceAxes=FollowerAxes  RotationSequence=XYX  RotationSequenceAngles=[0 0 0]  RotationSequenceAnglesUnits=deg  RotationMatrix=A01r
  A_01*E_1 : sm_lib/Frames and Transforms/Rigid Transform  TranslationMethod=Cartesian  TranslationStandardOffset=0  TranslationLengthUnit=mm  TranslationStandardAxis=+Z  TranslationCartesianOffset=A01t  TranslationROffset=0  TranslationROffsetUnits=m  TranslationZOffset=0  TranslationZOffsetUnits=m  TranslationThetaOffset=0  TranslationThetaOffsetUnits=deg  RotationMethod=None  RotationAngleUnits=deg  RotationStandardAxis=+Z  RotationAngle=0.0  RotationArbitraryAxis=[0 0 1]  FollAlignAxisA=+X  BaseAlignAxisA=+Y  FollAlignAxisB=+Y  BaseAlignAxisB=+Z  RotationSequenceAxes=FollowerAxes  RotationSequence=XYX  RotationSequenceAngles=[0 0 0]  RotationSequenceAnglesUnits=deg  RotationMatrix=A01r
  Mux : Mux  Inputs=3
  PS-Simulink Converter1 : nesl_utility/PS-Simulink Converter  PhysicalDomain=network_engine_domain  SubClassName=ps_output  LeftPortType=input  RightPortType=output  PseudoPeriodic=off  Frequencies=[]  Unit=1  AffineConversion=off
  PS-Simulink Converter2 : nesl_utility/PS-Simulink Converter  PhysicalDomain=network_engine_domain  SubClassName=ps_output  LeftPortType=input  RightPortType=output  PseudoPeriodic=off  Frequencies=[]  Unit=1  AffineConversion=off
  PS-Simulink Converter7 : nesl_utility/PS-Simulink Converter  PhysicalDomain=network_engine_domain  SubClassName=ps_output  LeftPortType=input  RightPortType=output  PseudoPeriodic=off  Frequencies=[]  Unit=1  AffineConversion=off
  Revolute Joint1 : sm_lib/Joints/Revolute Joint  JointMode=Normal  SenseConstraintForce=off  SenseConstraintForceX=off  SenseConstraintForceY=off  SenseConstraintForceZ=off  SenseConstraintTorque=off  SenseConstraintTorqueX=off  SenseConstraintTorqueY=off  SenseConstraintTorqueZ=off  SenseTotalForce=off  SenseTotalForceX=off  SenseTotalForceY=off  SenseTotalForceZ=off  SenseTotalTorque=off  SenseTotalTorqueX=off  SenseTotalTorqueY=off  SenseTotalTorqueZ=off  CompositeWrenchDir=FollowerOnBase  CompositeWrenchFrame=BaseFrame  EquilibriumPosition=0  EquilibriumPositionUnits=deg  SpringStiffness=0  SpringStiffnessUnits=N*m/deg  DampingCoefficient=0  DampingCoefficientUnits=N*m/(deg/s)  TorqueActuationMode=InputTorque  MotionActuationMode=ComputedMotion  SensePosition=on  SenseVelocity=on  SenseAcceleration=on  SenseTorqueForce=off  SenseLowerLimitTorqueForce=off  SenseUpperLimitTorqueForce=off  LowerLimitSpecify=on  LowerLimitBound=-J1.al  LowerLimitBoundUnits=deg  LowerLimitStiffness=1e4  LowerLimitStiffnessUnits=N*m/deg  LowerLimitDamping=10  LowerLimitDampingUnits=N*m/(deg/s)  LowerLimitTransitionRegionWidth=0.1  LowerLimitTransitionRegionWidthUnits=deg  UpperLimitSpecify=on  UpperLimitBound=J1.al  UpperLimitBoundUnits=deg  UpperLimitStiffness=1e4  UpperLimitStiffnessUnits=N*m/deg  UpperLimitDamping=10  UpperLimitDampingUnits=N*m/(deg/s)  UpperLimitTransitionRegionWidth=0.1  UpperLimitTransitionRegionWidthUnits=deg  PositionTargetSpecify=on  PositionTargetPriority=Low  PositionTargetValue=q0(1)  PositionTargetValueUnits=rad  VelocityTargetSpecify=off  VelocityTargetPriority=High  VelocityTargetValue=0  VelocityTargetValueUnits=deg/s
  Simulink-PS Converter : nesl_utility/Simulink-PS Converter  PhysicalDomain=network_engine_domain  SubClassName=ps_input  LeftPortType=input  RightPortType=output  PseudoPeriodic=off  Frequencies=[]  NoiseDistribution=none  NoiseParameters=[]  Unit=1  AffineConversion=off  FilteringAndDerivatives=provide  SimscapeFilterOrder=1  InputFilterTimeConstant=0.001  UdotUserProvided=0
  Link 0 : PMIOPort  Side=Left
  Link 1 : PMIOPort  Port=2  Side=Right
  q1,qd1,qdd1 : Outport
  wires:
  T1/1 -> Simulink-PS Converter/1
  PS-Simulink Converter7/1 -> Mux/2
  Mux/1 -> q1,qd1,qdd1/1
  PS-Simulink Converter1/1 -> Mux/1
  PS-Simulink Converter2/1 -> Mux/3
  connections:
  Revolute Joint1/LConn1 -- A_01*E_1/RConn1
  A_01*E_1/LConn1 -- A_01*E_01/RConn1
  Revolute Joint1/RConn1 -- Link 1/RConn1
  Link 0/RConn1 -- A_01*E_01/LConn1
  Simulink-PS Converter/RConn1 -- Revolute Joint1/LConn2
  Revolute Joint1/RConn2 -- PS-Simulink Converter1/LConn1
  Revolute Joint1/RConn3 -- PS-Simulink Converter7/LConn1
  Revolute Joint1/RConn4 -- PS-Simulink Converter2/LConn1

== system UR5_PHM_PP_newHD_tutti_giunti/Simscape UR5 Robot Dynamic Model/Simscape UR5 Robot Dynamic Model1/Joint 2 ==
  T2 : Inport
  A_12*E_1 : sm_lib/Frames and Transforms/Rigid Transform  TranslationMethod=Cartesian  TranslationStandardOffset=0  TranslationLengthUnit=mm  TranslationStandardAxis=+Z  TranslationCartesianOffset=A12t  TranslationROffset=0  TranslationROffsetUnits=m  TranslationZOffset=0  TranslationZOffsetUnits=m  TranslationThetaOffset=0  TranslationThetaOffsetUnits=deg  RotationMethod=None  RotationAngleUnits=deg  RotationStandardAxis=+Z  RotationAngle=0.0  RotationArbitraryAxis=[0 0 1]  FollAlignAxisA=+X  BaseAlignAxisA=+Y  FollAlignAxisB=+Y  BaseAlignAxisB=+Z  RotationSequenceAxes=FollowerAxes  RotationSequence=XYX  RotationSequenceAngles=[0 0 0]  RotationSequenceAnglesUnits=deg  RotationMatrix=A12r
  A_12*E_12 : sm_lib/Frames and Transforms/Rigid Transform  TranslationMethod=None  TranslationStandardOffset=0  TranslationLengthUnit=mm  TranslationStandardAxis=+Z  TranslationCartesianOffset=A12t  TranslationROffset=0  TranslationROffsetUnits=m  TranslationZOffset=0  TranslationZOffsetUnits=m  TranslationThetaOffset=0  TranslationThetaOffsetUnits=deg  RotationMethod=RotationMatrix  RotationAngleUnits=deg  RotationStandardAxis=+Z  RotationAngle=0.0  RotationArbitraryAxis=[0 0 1]  FollAlignAxisA=+X  BaseAlignAxisA=+Y  FollAlignAxisB=+Y  BaseAlignAxisB=+Z  RotationSequenceAxes=FollowerAxes  RotationSequence=XYX  RotationSequenceAngles=[0 0 0]  RotationSequenceAnglesUnits=deg  RotationMatrix=A12r
  Mux : Mux  Inputs=3
  PS-Simulink Converter1 : nesl_utility/PS-Simulink Converter  PhysicalDomain=network_engine_domain  SubClassName=ps_output  LeftPortType=input  RightPortType=output  PseudoPeriodic=off  Frequencies=[]  Unit=1  AffineConversion=off
  PS-Simulink Converter2 : nesl_utility/PS-Simulink Converter  PhysicalDomain=network_engine_domain  SubClassName=ps_output  LeftPortType=input  RightPortType=output  PseudoPeriodic=off  Frequencies=[]  Unit=1  AffineConversion=off
  PS-Simulink Converter7 : nesl_utility/PS-Simulink Converter  PhysicalDomain=network_engine_domain  SubClassName=ps_output  LeftPortType=input  RightPortType=output  PseudoPeriodic=off  Frequencies=[]  Unit=1  AffineConversion=off
  Revolute Joint2 : sm_lib/Joints/Revolute Joint  JointMode=Normal  SenseConstraintForce=off  SenseConstraintForceX=off  SenseConstraintForceY=off  SenseConstraintForceZ=off  SenseConstraintTorque=off  SenseConstraintTorqueX=off  SenseConstraintTorqueY=off  SenseConstraintTorqueZ=off  SenseTotalForce=off  SenseTotalForceX=off  SenseTotalForceY=off  SenseTotalForceZ=off  SenseTotalTorque=off  SenseTotalTorqueX=off  SenseTotalTorqueY=off  SenseTotalTorqueZ=off  CompositeWrenchDir=FollowerOnBase  CompositeWrenchFrame=BaseFrame  EquilibriumPosition=0  EquilibriumPositionUnits=deg  SpringStiffness=0  SpringStiffnessUnits=N*m/deg  DampingCoefficient=0  DampingCoefficientUnits=N*m/(deg/s)  TorqueActuationMode=InputTorque  MotionActuationMode=ComputedMotion  SensePosition=on  SenseVelocity=on  SenseAcceleration=on  SenseTorqueForce=off  SenseLowerLimitTorqueForce=off  SenseUpperLimitTorqueForce=off  LowerLimitSpecify=on  LowerLimitBound=-J2.al  LowerLimitBoundUnits=deg  LowerLimitStiffness=1e4  LowerLimitStiffnessUnits=N*m/deg  LowerLimitDamping=10  LowerLimitDampingUnits=N*m/(deg/s)  LowerLimitTransitionRegionWidth=0.1  LowerLimitTransitionRegionWidthUnits=deg  UpperLimitSpecify=on  UpperLimitBound=J2.al  UpperLimitBoundUnits=deg  UpperLimitStiffness=1e4  UpperLimitStiffnessUnits=N*m/deg  UpperLimitDamping=10  UpperLimitDampingUnits=N*m/(deg/s)  UpperLimitTransitionRegionWidth=0.1  UpperLimitTransitionRegionWidthUnits=deg  PositionTargetSpecify=on  PositionTargetPriority=High  PositionTargetValue=q0(2)  PositionTargetValueUnits=rad  VelocityTargetSpecify=off  VelocityTargetPriority=High  VelocityTargetValue=0  VelocityTargetValueUnits=deg/s
  Simulink-PS Converter : nesl_utility/Simulink-PS Converter  PhysicalDomain=network_engine_domain  SubClassName=ps_input  LeftPortType=input  RightPortType=output  PseudoPeriodic=off  Frequencies=[]  NoiseDistribution=none  NoiseParameters=[]  Unit=1  AffineConversion=off  FilteringAndDerivatives=provide  SimscapeFilterOrder=1  InputFilterTimeConstant=0.001  UdotUserProvided=0
  Link 1 : PMIOPort  Side=Left
  Link 2 : PMIOPort  Port=2  Side=Right
  q2,qd2,qdd2 : Outport
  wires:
  PS-Simulink Converter1/1 -> Mux/1
  T2/1 -> Simulink-PS Converter/1
  Mux/1 -> q2,qd2,qdd2/1
  PS-Simulink Converter7/1 -> Mux/2
  PS-Simulink Converter2/1 -> Mux/3
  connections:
  Revolute Joint2/LConn1 -- A_12*E_1/RConn1
  A_12*E_1/LConn1 -- A_12*E_12/RConn1
  Revolute Joint2/RConn1 -- Link 2/RConn1
  A_12*E_12/LConn1 -- Link 1/RConn1
  Revolute Joint2/RConn4 -- PS-Simulink Converter2/LConn1
  Revolute Joint2/LConn2 -- Simulink-PS Converter/RConn1
  Revolute Joint2/RConn3 -- PS-Simulink Converter7/LConn1
  Revolute Joint2/RConn2 -- PS-Simulink Converter1/LConn1

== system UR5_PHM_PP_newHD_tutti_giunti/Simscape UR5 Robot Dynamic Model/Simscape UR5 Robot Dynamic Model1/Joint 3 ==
  T3 : Inport
  A_23*E_1 : sm_lib/Frames and Transforms/Rigid Transform  TranslationMethod=Cartesian  TranslationStandardOffset=0  TranslationLengthUnit=mm  TranslationStandardAxis=+Z  TranslationCartesianOffset=A23t  TranslationROffset=0  TranslationROffsetUnits=m  TranslationZOffset=0  TranslationZOffsetUnits=m  TranslationThetaOffset=0  TranslationThetaOffsetUnits=deg  RotationMethod=None  RotationAngleUnits=deg  RotationStandardAxis=+Z  RotationAngle=0.0  RotationArbitraryAxis=[0 0 1]  FollAlignAxisA=+X  BaseAlignAxisA=+Y  FollAlignAxisB=+Y  BaseAlignAxisB=+Z  RotationSequenceAxes=FollowerAxes  RotationSequence=XYX  RotationSequenceAngles=[0 0 0]  RotationSequenceAnglesUnits=deg  RotationMatrix=A23r
  A_23*E_23 : sm_lib/Frames and Transforms/Rigid Transform  TranslationMethod=None  TranslationStandardOffset=0  TranslationLengthUnit=mm  TranslationStandardAxis=+Z  TranslationCartesianOffset=A23t  TranslationROffset=0  TranslationROffsetUnits=m  TranslationZOffset=0  TranslationZOffsetUnits=m  TranslationThetaOffset=0  TranslationThetaOffsetUnits=deg  RotationMethod=RotationMatrix  RotationAngleUnits=deg  RotationStandardAxis=+Z  RotationAngle=0.0  RotationArbitraryAxis=[0 0 1]  FollAlignAxisA=+X  BaseAlignAxisA=+Y  FollAlignAxisB=+Y  BaseAlignAxisB=+Z  RotationSequenceAxes=FollowerAxes  RotationSequence=XYX  RotationSequenceAngles=[0 0 0]  RotationSequenceAnglesUnits=deg  RotationMatrix=A23r
  Mux : Mux  Inputs=3
  PS-Simulink Converter1 : nesl_utility/PS-Simulink Converter  PhysicalDomain=network_engine_domain  SubClassName=ps_output  LeftPortType=input  RightPortType=output  PseudoPeriodic=off  Frequencies=[]  Unit=1  AffineConversion=off
  PS-Simulink Converter2 : nesl_utility/PS-Simulink Converter  PhysicalDomain=network_engine_domain  SubClassName=ps_output  LeftPortType=input  RightPortType=output  PseudoPeriodic=off  Frequencies=[]  Unit=1  AffineConversion=off
  PS-Simulink Converter7 : nesl_utility/PS-Simulink Converter  PhysicalDomain=network_engine_domain  SubClassName=ps_output  LeftPortType=input  RightPortType=output  PseudoPeriodic=off  Frequencies=[]  Unit=1  AffineConversion=off
  Revolute Joint3 : sm_lib/Joints/Revolute Joint  JointMode=Normal  SenseConstraintForce=off  SenseConstraintForceX=off  SenseConstraintForceY=off  SenseConstraintForceZ=off  SenseConstraintTorque=off  SenseConstraintTorqueX=off  SenseConstraintTorqueY=off  SenseConstraintTorqueZ=off  SenseTotalForce=off  SenseTotalForceX=off  SenseTotalForceY=off  SenseTotalForceZ=off  SenseTotalTorque=off  SenseTotalTorqueX=off  SenseTotalTorqueY=off  SenseTotalTorqueZ=off  CompositeWrenchDir=FollowerOnBase  CompositeWrenchFrame=BaseFrame  EquilibriumPosition=0  EquilibriumPositionUnits=deg  SpringStiffness=0  SpringStiffnessUnits=N*m/deg  DampingCoefficient=0  DampingCoefficientUnits=N*m/(deg/s)  TorqueActuationMode=InputTorque  MotionActuationMode=ComputedMotion  SensePosition=on  SenseVelocity=on  SenseAcceleration=on  SenseTorqueForce=off  SenseLowerLimitTorqueForce=off  SenseUpperLimitTorqueForce=off  LowerLimitSpecify=on  LowerLimitBound=-J3.al  LowerLimitBoundUnits=deg  LowerLimitStiffness=1e4  LowerLimitStiffnessUnits=N*m/deg  LowerLimitDamping=10  LowerLimitDampingUnits=N*m/(deg/s)  LowerLimitTransitionRegionWidth=0.1  LowerLimitTransitionRegionWidthUnits=deg  UpperLimitSpecify=on  UpperLimitBound=J3.al  UpperLimitBoundUnits=deg  UpperLimitStiffness=1e4  UpperLimitStiffnessUnits=N*m/deg  UpperLimitDamping=10  UpperLimitDampingUnits=N*m/(deg/s)  UpperLimitTransitionRegionWidth=0.1  UpperLimitTransitionRegionWidthUnits=deg  PositionTargetSpecify=on  PositionTargetPriority=Low  PositionTargetValue=q0(3)  PositionTargetValueUnits=rad  VelocityTargetSpecify=off  VelocityTargetPriority=High  VelocityTargetValue=0  VelocityTargetValueUnits=deg/s
  Simulink-PS Converter : nesl_utility/Simulink-PS Converter  PhysicalDomain=network_engine_domain  SubClassName=ps_input  LeftPortType=input  RightPortType=output  PseudoPeriodic=off  Frequencies=[]  NoiseDistribution=none  NoiseParameters=[]  Unit=1  AffineConversion=off  FilteringAndDerivatives=provide  SimscapeFilterOrder=1  InputFilterTimeConstant=0.001  UdotUserProvided=0
  Link 2 : PMIOPort  Side=Left
  Link 3 : PMIOPort  Port=2  Side=Right
  q3,qd3,qdd3 : Outport
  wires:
  PS-Simulink Converter1/1 -> Mux/1
  T3/1 -> Simulink-PS Converter/1
  Mux/1 -> q3,qd3,qdd3/1
  PS-Simulink Converter7/1 -> Mux/2
  PS-Simulink Converter2/1 -> Mux/3
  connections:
  A_23*E_1/RConn1 -- Revolute Joint3/LConn1
  A_23*E_1/LConn1 -- A_23*E_23/RConn1
  A_23*E_23/LConn1 -- Link 2/RConn1
  Revolute Joint3/RConn1 -- Link 3/RConn1
  Revolute Joint3/RConn4 -- PS-Simulink Converter2/LConn1
  Revolute Joint3/LConn2 -- Simulink-PS Converter/RConn1
  Revolute Joint3/RConn3 -- PS-Simulink Converter7/LConn1
  Revolute Joint3/RConn2 -- PS-Simulink Converter1/LConn1

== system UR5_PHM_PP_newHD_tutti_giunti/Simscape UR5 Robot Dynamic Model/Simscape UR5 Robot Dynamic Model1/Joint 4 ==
  T4 : Inport
  A_34*E_1 : sm_lib/Frames and Transforms/Rigid Transform  TranslationMethod=Cartesian  TranslationStandardOffset=0  TranslationLengthUnit=mm  TranslationStandardAxis=+Z  TranslationCartesianOffset=A34t  TranslationROffset=0  TranslationROffsetUnits=m  TranslationZOffset=0  TranslationZOffsetUnits=m  TranslationThetaOffset=0  TranslationThetaOffsetUnits=deg  RotationMethod=None  RotationAngleUnits=deg  RotationStandardAxis=+Z  RotationAngle=0.0  RotationArbitraryAxis=[0 0 1]  FollAlignAxisA=+X  BaseAlignAxisA=+Y  FollAlignAxisB=+Y  BaseAlignAxisB=+Z  RotationSequenceAxes=FollowerAxes  RotationSequence=XYX  RotationSequenceAngles=[0 0 0]  RotationSequenceAnglesUnits=deg  RotationMatrix=A34r
  A_34*E_34 : sm_lib/Frames and Transforms/Rigid Transform  TranslationMethod=None  TranslationStandardOffset=0  TranslationLengthUnit=mm  TranslationStandardAxis=+Z  TranslationCartesianOffset=A34t  TranslationROffset=0  TranslationROffsetUnits=m  TranslationZOffset=0  TranslationZOffsetUnits=m  TranslationThetaOffset=0  TranslationThetaOffsetUnits=deg  RotationMethod=RotationMatrix  RotationAngleUnits=deg  RotationStandardAxis=+Z  RotationAngle=0.0  RotationArbitraryAxis=[0 0 1]  FollAlignAxisA=+X  BaseAlignAxisA=+Y  FollAlignAxisB=+Y  BaseAlignAxisB=+Z  RotationSequenceAxes=FollowerAxes  RotationSequence=XYX  RotationSequenceAngles=[0 0 0]  RotationSequenceAnglesUnits=deg  RotationMatrix=A34r
  Mux : Mux  Inputs=3
  PS-Simulink Converter1 : nesl_utility/PS-Simulink Converter  PhysicalDomain=network_engine_domain  SubClassName=ps_output  LeftPortType=input  RightPortType=output  PseudoPeriodic=off  Frequencies=[]  Unit=1  AffineConversion=off
  PS-Simulink Converter2 : nesl_utility/PS-Simulink Converter  PhysicalDomain=network_engine_domain  SubClassName=ps_output  LeftPortType=input  RightPortType=output  PseudoPeriodic=off  Frequencies=[]  Unit=1  AffineConversion=off
  PS-Simulink Converter7 : nesl_utility/PS-Simulink Converter  PhysicalDomain=network_engine_domain  SubClassName=ps_output  LeftPortType=input  RightPortType=output  PseudoPeriodic=off  Frequencies=[]  Unit=1  AffineConversion=off
  Revolute Joint4 : sm_lib/Joints/Revolute Joint  JointMode=Normal  SenseConstraintForce=off  SenseConstraintForceX=off  SenseConstraintForceY=off  SenseConstraintForceZ=off  SenseConstraintTorque=off  SenseConstraintTorqueX=off  SenseConstraintTorqueY=off  SenseConstraintTorqueZ=off  SenseTotalForce=off  SenseTotalForceX=off  SenseTotalForceY=off  SenseTotalForceZ=off  SenseTotalTorque=off  SenseTotalTorqueX=off  SenseTotalTorqueY=off  SenseTotalTorqueZ=off  CompositeWrenchDir=FollowerOnBase  CompositeWrenchFrame=BaseFrame  EquilibriumPosition=0  EquilibriumPositionUnits=deg  SpringStiffness=0  SpringStiffnessUnits=N*m/deg  DampingCoefficient=0  DampingCoefficientUnits=N*m/(deg/s)  TorqueActuationMode=InputTorque  MotionActuationMode=ComputedMotion  SensePosition=on  SenseVelocity=on  SenseAcceleration=on  SenseTorqueForce=off  SenseLowerLimitTorqueForce=off  SenseUpperLimitTorqueForce=off  LowerLimitSpecify=on  LowerLimitBound=-J4.al  LowerLimitBoundUnits=deg  LowerLimitStiffness=1e4  LowerLimitStiffnessUnits=N*m/deg  LowerLimitDamping=10  LowerLimitDampingUnits=N*m/(deg/s)  LowerLimitTransitionRegionWidth=0.1  LowerLimitTransitionRegionWidthUnits=deg  UpperLimitSpecify=on  UpperLimitBound=J4.al  UpperLimitBoundUnits=deg  UpperLimitStiffness=1e4  UpperLimitStiffnessUnits=N*m/deg  UpperLimitDamping=10  UpperLimitDampingUnits=N*m/(deg/s)  UpperLimitTransitionRegionWidth=0.1  UpperLimitTransitionRegionWidthUnits=deg  PositionTargetSpecify=on  PositionTargetPriority=Low  PositionTargetValue=q0(4)  PositionTargetValueUnits=rad  VelocityTargetSpecify=off  VelocityTargetPriority=High  VelocityTargetValue=0  VelocityTargetValueUnits=deg/s
  Simulink-PS Converter : nesl_utility/Simulink-PS Converter  PhysicalDomain=network_engine_domain  SubClassName=ps_input  LeftPortType=input  RightPortType=output  PseudoPeriodic=off  Frequencies=[]  NoiseDistribution=none  NoiseParameters=[]  Unit=1  AffineConversion=off  FilteringAndDerivatives=provide  SimscapeFilterOrder=1  InputFilterTimeConstant=0.001  UdotUserProvided=0
  Link 3 : PMIOPort  Side=Left
  Link 4 : PMIOPort  Port=2  Side=Right
  q4,qd4,qdd4 : Outport
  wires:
  PS-Simulink Converter1/1 -> Mux/1
  T4/1 -> Simulink-PS Converter/1
  Mux/1 -> q4,qd4,qdd4/1
  PS-Simulink Converter7/1 -> Mux/2
  PS-Simulink Converter2/1 -> Mux/3
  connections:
  A_34*E_1/LConn1 -- A_34*E_34/RConn1
  A_34*E_1/RConn1 -- Revolute Joint4/LConn1
  Link 3/RConn1 -- A_34*E_34/LConn1
  Revolute Joint4/RConn1 -- Link 4/RConn1
  Revolute Joint4/RConn4 -- PS-Simulink Converter2/LConn1
  Revolute Joint4/LConn2 -- Simulink-PS Converter/RConn1
  Revolute Joint4/RConn3 -- PS-Simulink Converter7/LConn1
  Revolute Joint4/RConn2 -- PS-Simulink Converter1/LConn1
